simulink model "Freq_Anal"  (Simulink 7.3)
settings: Solver=ode45  StartTime=0.0  StopTime=20  RelTol=1e-3
undefined symbols (not defined in the file or in its folder): Ali, Bli, Cli, Dli, Kpr

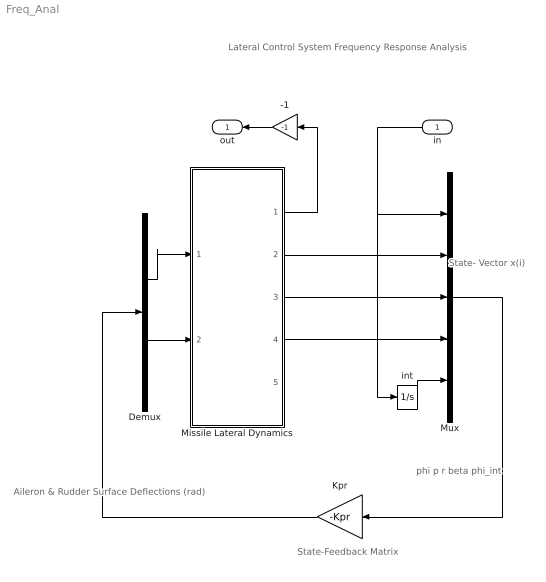
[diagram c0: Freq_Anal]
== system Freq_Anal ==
  note: phi p r beta phi_int
  note: State- Vector x(i)
  note: Aileron & Rudder Surface Deflections (rad)
  note: State-Feedback Matrix
  note: Lateral Control System Frequency Response Analysis
  in : Inport  OutDataType=sfix(16)  OutScaling=2^0
  -1 : Gain  Gain=-1  ParameterDataType=fixdt(1, 16)  ParameterScaling=2^0  OutDataType=fixdt(1, 16)  OutScaling=2^0
  Demux : Demux  Outputs=2
  Kpr : Gain  Gain=-Kpr  Multiplication=Matrix(K*u)  ParameterDataType=fixdt(1, 16)  ParameterScaling=2^0  OutDataType=fixdt(1, 16)  OutScaling=2^0
  Missile Lateral Dynamics : Subsystem
  Mux : Mux  Inputs=5
  int : Integrator
  out : Outport  OutDataType=sfix(16)  OutScaling=2^0
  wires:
  Demux/2 -> Missile Lateral Dynamics/2(rudd)
  Kpr/1 -> Demux/1
  Mux/1 -> Kpr/1
  Demux/1 -> Missile Lateral Dynamics/1(ailer)
  Missile Lateral Dynamics/2(p) -> Mux/2
  Missile Lateral Dynamics/3(r) -> Mux/3
  Missile Lateral Dynamics/4(beta) -> Mux/4
  Missile Lateral Dynamics/1(phi) -> -1/1
  in/1 -> Mux/1, int/1
  int/1 -> Mux/5
  -1/1 -> out/1

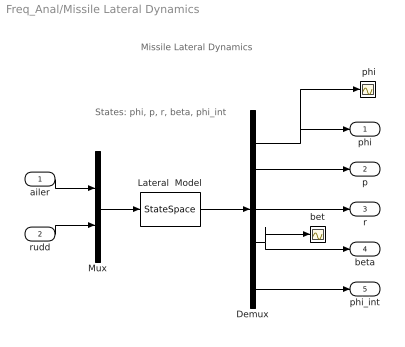
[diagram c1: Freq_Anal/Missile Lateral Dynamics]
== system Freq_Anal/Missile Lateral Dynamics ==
  note: Missile Lateral Dynamics
  note: States: phi, p, r, beta, phi_int
  ailer : Inport  OutDataType=sfix(16)  OutScaling=2^0
  rudd : Inport  Port=2  OutDataType=sfix(16)  OutScaling=2^0
  " phi" : Scope
  Demux : Demux  Outputs=5
  Lateral  Model : StateSpace  A=Ali  B=Bli  C=Cli  D=Dli
  Mux : Mux  Inputs=2
  bet : Scope
  phi : Outport  OutDataType=sfix(16)  OutScaling=2^0
  p : Outport  Port=2  OutDataType=sfix(16)  OutScaling=2^0
  r : Outport  Port=3  OutDataType=sfix(16)  OutScaling=2^0
  beta : Outport  Port=4  OutDataType=sfix(16)  OutScaling=2^0
  phi_int : Outport  Port=5  OutDataType=sfix(16)  OutScaling=2^0
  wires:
  Mux/1 -> Lateral  Model/1
  Lateral  Model/1 -> Demux/1
  ailer/1 -> Mux/1
  rudd/1 -> Mux/2
  Demux/1 -> phi/1, " phi"/1
  Demux/2 -> p/1
  Demux/3 -> r/1
  Demux/4 -> beta/1, bet/1
  Demux/5 -> phi_int/1
